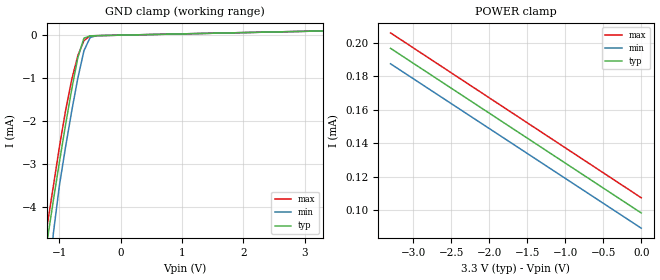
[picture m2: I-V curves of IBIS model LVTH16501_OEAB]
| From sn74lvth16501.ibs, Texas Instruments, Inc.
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|   LVTH16501 Input (OEAB) model
[Model]   LVTH16501_OEAB
Model_type  Input
Polarity   Non-Inverting
Vinl = 0.8V
Vinh = 2.0V
| variable   typ   min   max
C_comp   3.5p   NA   NA
[Temperature Range]   50   100   0
[Voltage range]   3.3   3   3.6
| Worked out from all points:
|   GND clamp passes 1 mA (typ) near -0.76 V on its own axis
|Process range|   weak   strong
[GND Clamp]
|   50C:3.3V:   100C:3V:weak   0C:3.6V:strong
|   Voltage   I(typ)   I(min)   I(max)
-3.3V     -71.52mA   -75.94mA   -67.21mA
-1.3V     -5.975mA   -8.539mA   -5.385mA
-1.2V     -4.793mA   -6.306mA   -4.435mA
-1.1V     -3.853mA   -4.622mA   -3.522mA
-1V       -2.951mA   -3.494mA   -2.597mA
-900mV    -2.086mA   -2.602mA   -1.758mA
-800mV    -1.262mA   -1.77mA    -1.033mA
-700mV    -520.9uA   -1mA       -479.6uA
-600mV    -69.9uA    -361.8uA   -125.3uA
-500mV    -16.62uA   -56.9uA    -15.76uA
-400mV    -11.97uA   -14.08uA   -11.95uA
3.3V      98.36uA    98.2uA     98.49uA
[POWER Clamp]
|   50C:3.3V:   100C:3V:weak   0C:3.6V:strong
|   Voltage   I(typ)   I(min)   I(max)
-3.3V     196.7uA    187.5uA    205.9uA
-1.9V     155uA      145.8uA    164.2uA
-100mV    101.3uA    92.25uA    110.4uA
0V        98.36uA    89.27uA    107.4uA
